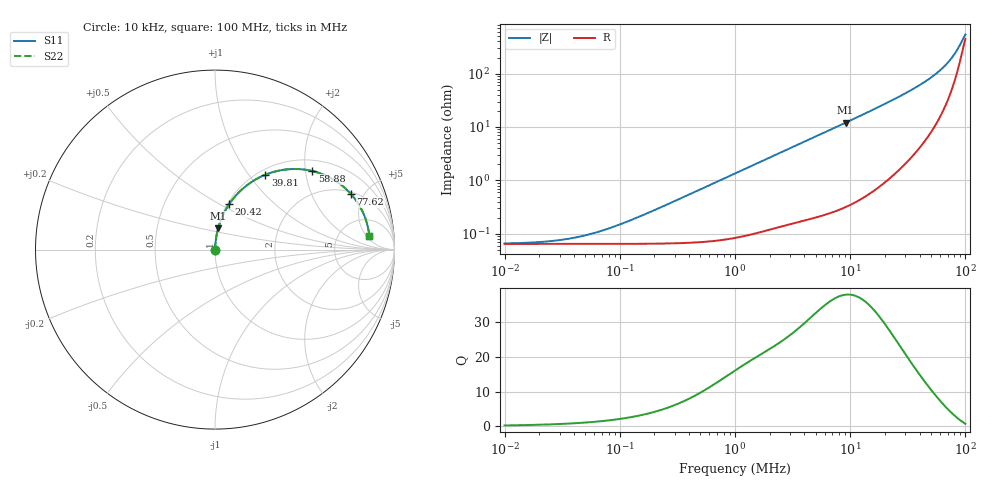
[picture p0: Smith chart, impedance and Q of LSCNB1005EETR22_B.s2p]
! LSCNB1005EETR22_B  S-PARAMETER MODEL  ( Standard Model )
! Model Generated by TAIYO YUDEN Corporation (http://www.ty-top.com)
! Version 1.0
! TAIYO YUDEN Control No. 190130
! Copyright(c) 2019 TAIYO YUDEN CO.,LTD. All Rights Reserved.
! Product Description (link to TY-COMPAS)
! https://ds.yuden.co.jp/TYCOMPAS/or/detail?pn=LSCNB1005EETR22MB&u=M
! Products Name : Inductors
! Characteristics :
!  Inductance : 0.22 [uH] , SRF(min) : - [Hz] , DC Resistance(max) : 80 [mOhm]
!  Rated Current : Saturation  1.6 [A] (dL = 30 [%]), Temp Rise  1.6 [A] (dT = 40 [degC])
!  Case Size : 1.0 x 0.5 / 0.039 x 0.02 [mm/inch] , Thickness : 0.55 / 0.022 [mm/inch]
!  (Conditions: Temperature = 25 [degC] , DC Bias Current = 0 [A])
! External Node Assignments :
!  1  o---GGG---o  2
! GND o---------o GND
! Frequency Range : 10kHz  -  100MHz  [ 402 STEP ]
# MHz S RI R 50
! Freq[MHz].  S11 Real  S11 Imag  S21 Real  S21 Imag  S12 Real  S12 Imag  S22 Real  S22 Imag
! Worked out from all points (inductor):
!   401 points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, 10 kHz to 100 MHz, reference 50 ohm
!   read as one part in series: L = 216 nH near 144.5 kHz
!   highest Q = 37.9 at 9.12 MHz (marker M1), where L = 210 nH
!   S11 on the Smith chart (normalised r, x): 10 kHz: 1.00, +0.00; 20.42 MHz: 1.02, +0.55; 39.81 MHz: 1.08, +1.21; 58.88 MHz: 1.28, +2.18; 77.62 MHz: 2.13, +4.00; 100 MHz: 10, +6
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0.01  0.00065 0.000135  0.9994 -0.000135  0.9994 -0.000135  0.00065 0.000135
0.023988  0.00065 0.000324  0.9994 -0.000324  0.9994 -0.000324  0.00065 0.000324
0.033884  0.00065 0.000458  0.9994 -0.000458  0.9994 -0.000458  0.00065 0.000458
0.046774  0.00065 0.000633  0.9993 -0.000633  0.9993 -0.000633  0.00065 0.000633
0.064565  0.000651 0.000874  0.9993 -0.000874  0.9993 -0.000874  0.000651 0.000874
0.091201  0.000652 0.00123  0.9993 -0.00123  0.9993 -0.00123  0.000652 0.00123
0.218776  0.000667 0.00296  0.9993 -0.00296  0.9993 -0.00296  0.000667 0.00296
1  0.00102 0.0135  0.999 -0.0135  0.999 -0.0135  0.00102 0.0135
4.677351  0.00572 0.0613  0.9943 -0.0613  0.9943 -0.0613  0.00572 0.0613
9.120108  0.0173 0.1179  0.9827 -0.1179  0.9827 -0.1179  0.0173 0.1179
14.4544  0.0407 0.1838  0.9593 -0.1838  0.9593 -0.1838  0.0407 0.1838
20.41738  0.0788 0.2528  0.9212 -0.2528  0.9212 -0.2528  0.0788 0.2528
21.87762  0.09 0.2687  0.91 -0.2687  0.91 -0.2687  0.09 0.2687
30.19952  0.1671 0.3497  0.8329 -0.3497  0.8329 -0.3497  0.1671 0.3497
39.81072  0.2803 0.417  0.7197 -0.417  0.7197 -0.417  0.2803 0.417
48.97788  0.4044 0.4474  0.5956 -0.4474  0.5956 -0.4474  0.4044 0.4474
58.88437  0.5427 0.4377  0.4573 -0.4377  0.4573 -0.4377  0.5427 0.4377
67.6083  0.6547 0.3933  0.3453 -0.3933  0.3453 -0.3933  0.6547 0.3933
77.62471  0.7574 0.3097  0.2426 -0.3097  0.2426 -0.3097  0.7574 0.3097
89.12509  0.8312 0.1911  0.1688 -0.1911  0.1688 -0.1911  0.8312 0.1911
95.49926  0.8522 0.1237  0.1478 -0.1237  0.1478 -0.1237  0.8522 0.1237
100  0.86 0.0776  0.14 -0.0776  0.14 -0.0776  0.86 0.0776
